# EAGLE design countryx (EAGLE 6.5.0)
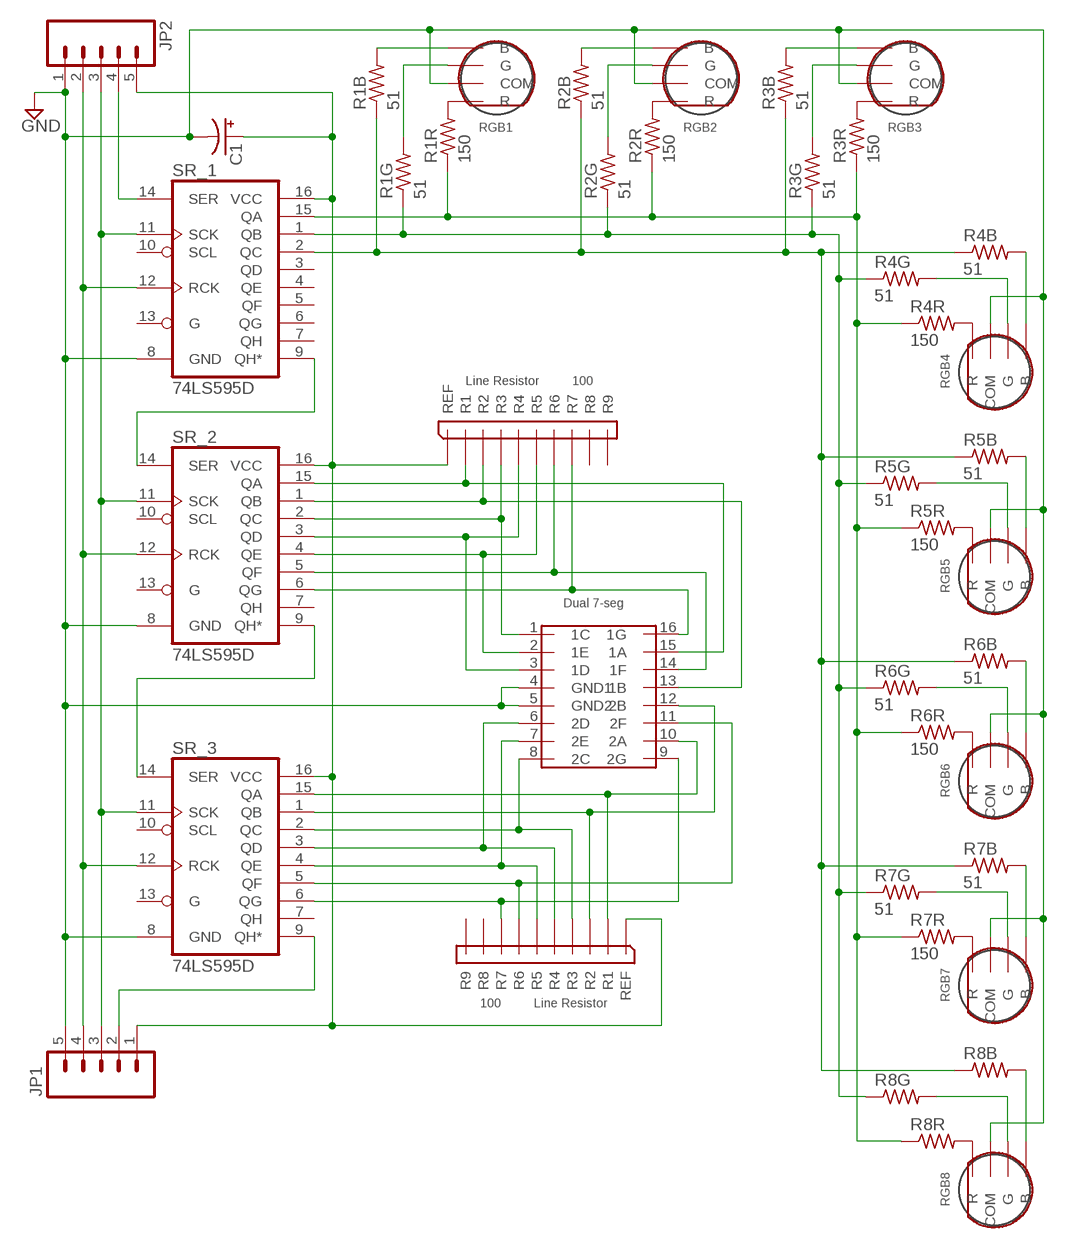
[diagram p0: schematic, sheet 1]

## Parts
C1  CPOL-USE2,5-6E  [E2,5-6E]
JP1  M05LOCK  [1X05_LOCK]
JP2  M05LOCK  [1X05_LOCK]
R1B  51  R-US_0204/5  [0204/5]
R1G  51  R-US_0204/5  [0204/5]
R1R  150  R-US_0204/5  [0204/5]
R2B  51  R-US_0204/5  [0204/5]
R2G  51  R-US_0204/5  [0204/5]
R2R  150  R-US_0204/5  [0204/5]
R3B  51  R-US_0204/5  [0204/5]
R3G  51  R-US_0204/5  [0204/5]
R3R  150  R-US_0204/5  [0204/5]
R4B  51  R-US_0204/5  [0204/5]
R4G  51  R-US_0204/5  [0204/5]
R4R  150  R-US_0204/5  [0204/5]
R5B  51  R-US_0204/5  [0204/5]
R5G  51  R-US_0204/5  [0204/5]
R5R  150  R-US_0204/5  [0204/5]
R6B  51  R-US_0204/5  [0204/5]
R6G  51  R-US_0204/5  [0204/5]
R6R  150  R-US_0204/5  [0204/5]
R7B  51  R-US_0204/5  [0204/5]
R7G  51  R-US_0204/5  [0204/5]
R7R  150  R-US_0204/5  [0204/5]
R8B  R-US_R0805  [R0805]
R8G  R-US_R0805  [R0805]
R8R  R-US_R0805  [R0805]
RGB1  RGBLED  [3LED]
RGB2  RGBLED  [3LED]
RGB3  RGBLED  [3LED]
RGB4  RGBLED  [3LED]
RGB5  RGBLED  [3LED]
RGB6  RGBLED  [3LED]
RGB7  RGBLED  [3LED]
RGB8  RGBLED  [3LED]
SR_1  74LS595D  [SO16]
SR_2  74LS595D  [SO16]
SR_3  74LS595D  [SO16]
U$1  HDSP-G03E  [HDSP-G]
U$2  100  4610X  [4610X]
U$3  100  4610X  [4610X]

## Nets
GND: C1.- JP1.5 JP2.1 RGB1.COM RGB2.COM RGB3.COM RGB4.COM RGB5.COM RGB6.COM RGB7.COM RGB8.COM SR_1.8(GND) SR_2.8(GND) SR_3.8(GND) U$1.4(GND1) U$1.5(GND2)
N$1: R1R.1 R2R.1 R3R.1 R4R.1 R5R.1 R6R.1 R7R.1 R8R.1 SR_1.15(QA)
N$2: R1B.1 R2B.1 R3B.1 R4B.1 R5B.1 R6B.1 R7B.1 R8B.1 SR_1.2(QC)
N$3: R8R.2 RGB8.R
N$4: SR_2.15(QA) U$1.15(1A) U$2.R1
N$5: SR_2.1(QB) U$1.13(1B) U$2.R2
N$6: SR_2.2(QC) U$1.1(1C) U$2.R3
N$7: SR_2.3(QD) U$1.3(1D) U$2.R4
N$8: R1R.2 RGB1.R
N$9: SR_2.5(QF) U$1.14(1F) U$2.R6
N$10: SR_2.6(QG) U$1.16(1G) U$2.R7
N$11: SR_3.6(QG) U$1.9(2G) U$3.R7
N$12: SR_3.5(QF) U$1.11(2F) U$3.R6
N$13: SR_3.4(QE) U$1.7(2E) U$3.R5
N$14: SR_3.3(QD) U$1.6(2D) U$3.R4
N$15: SR_3.2(QC) U$1.8(2C) U$3.R3
N$16: SR_2.4(QE) U$1.2(1E) U$2.R5
N$17: SR_3.15(QA) U$1.10(2A) U$3.R1
N$18: R2R.2 RGB2.R
N$19: SR_3.1(QB) U$1.12(2B) U$3.R2
N$20: R3R.2 RGB3.R
N$25: R1G.2 RGB1.G
N$26: R2G.2 RGB2.G
N$27: R3G.2 RGB3.G
N$28: R1B.2 RGB1.B
N$29: R2B.2 RGB2.B
N$30: R3B.2 RGB3.B
N$32: R1G.1 R2G.1 R3G.1 R4G.1 R5G.1 R6G.1 R7G.1 R8G.1 SR_1.1(QB)
N$34: R4G.2 RGB4.G
N$35: R4B.2 RGB4.B
N$36: R4R.2 RGB4.R
N$39: R5G.2 RGB5.G
N$40: R5B.2 RGB5.B
N$41: R5R.2 RGB5.R
N$43: R6G.2 RGB6.G
N$44: R6B.2 RGB6.B
N$45: R6R.2 RGB6.R
N$46: R8G.2 RGB8.G
N$47: R8B.2 RGB8.B
N$49: R7G.2 RGB7.G
N$50: R7B.2 RGB7.B
N$51: R7R.2 RGB7.R
RCLK: JP1.4 JP2.2 SR_1.12(RCK) SR_2.12(RCK) SR_3.12(RCK)
SCLK: JP1.3 JP2.3 SR_1.11(SCK) SR_2.11(SCK) SR_3.11(SCK)
SER_12: SR_1.9(QH*) SR_2.14(SER)
SER_23: SR_2.9(QH*) SR_3.14(SER)
SER_IN: JP2.4 SR_1.14(SER)
SER_OUT: JP1.2 SR_3.9(QH*)
VCC: C1.+ JP1.1 JP2.5 SR_1.16(VCC) SR_2.16(VCC) SR_3.16(VCC) U$2.REF U$3.REF
Unconnected: SR_1.3(QD) SR_1.4(QE) SR_1.5(QF) SR_1.6(QG) SR_1.7(QH) SR_1.10(SCL) SR_1.13(G) SR_2.7(QH) SR_2.10(SCL) SR_2.13(G) SR_3.7(QH) SR_3.10(SCL) SR_3.13(G) U$2.R8 U$2.R9 U$3.R8 U$3.R9

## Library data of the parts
C1 = Power Supply:CPOL-US: POLARIZED CAPACITOR, American symbol
JP1 JP2 = SparkFun-Connectors:M05: Header 5 Standard 5-pin 0.1" header. Use with straight break away headers (SKU : PRT-00116), right angle break away headers (PRT-00553), swiss pins (PRT-00743), machine pins (PRT-00117), and female headers (PRT-00115). Molex polarized connector foot print use with SKU : PRT-08230 with associated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
R1B R1G R1R R2B R2G R2R R3B R3G R3R R4B R4G R4R R5B R5G R5R R6B R6G R6R R7B R7G R7R R8B R8G R8R = resistor:R-US_: RESISTOR, American symbol
RGB1-RGB8 = RISK:RGBLED
SR_1-SR_3 = SparkFun-DigitalIC:74*595: 8-bit SHIFT REGISTER, output latch; PROD_ID: IC-07875
U$1 = RISK:HDSP-G03E
U$2 U$3 = RISK:4610X

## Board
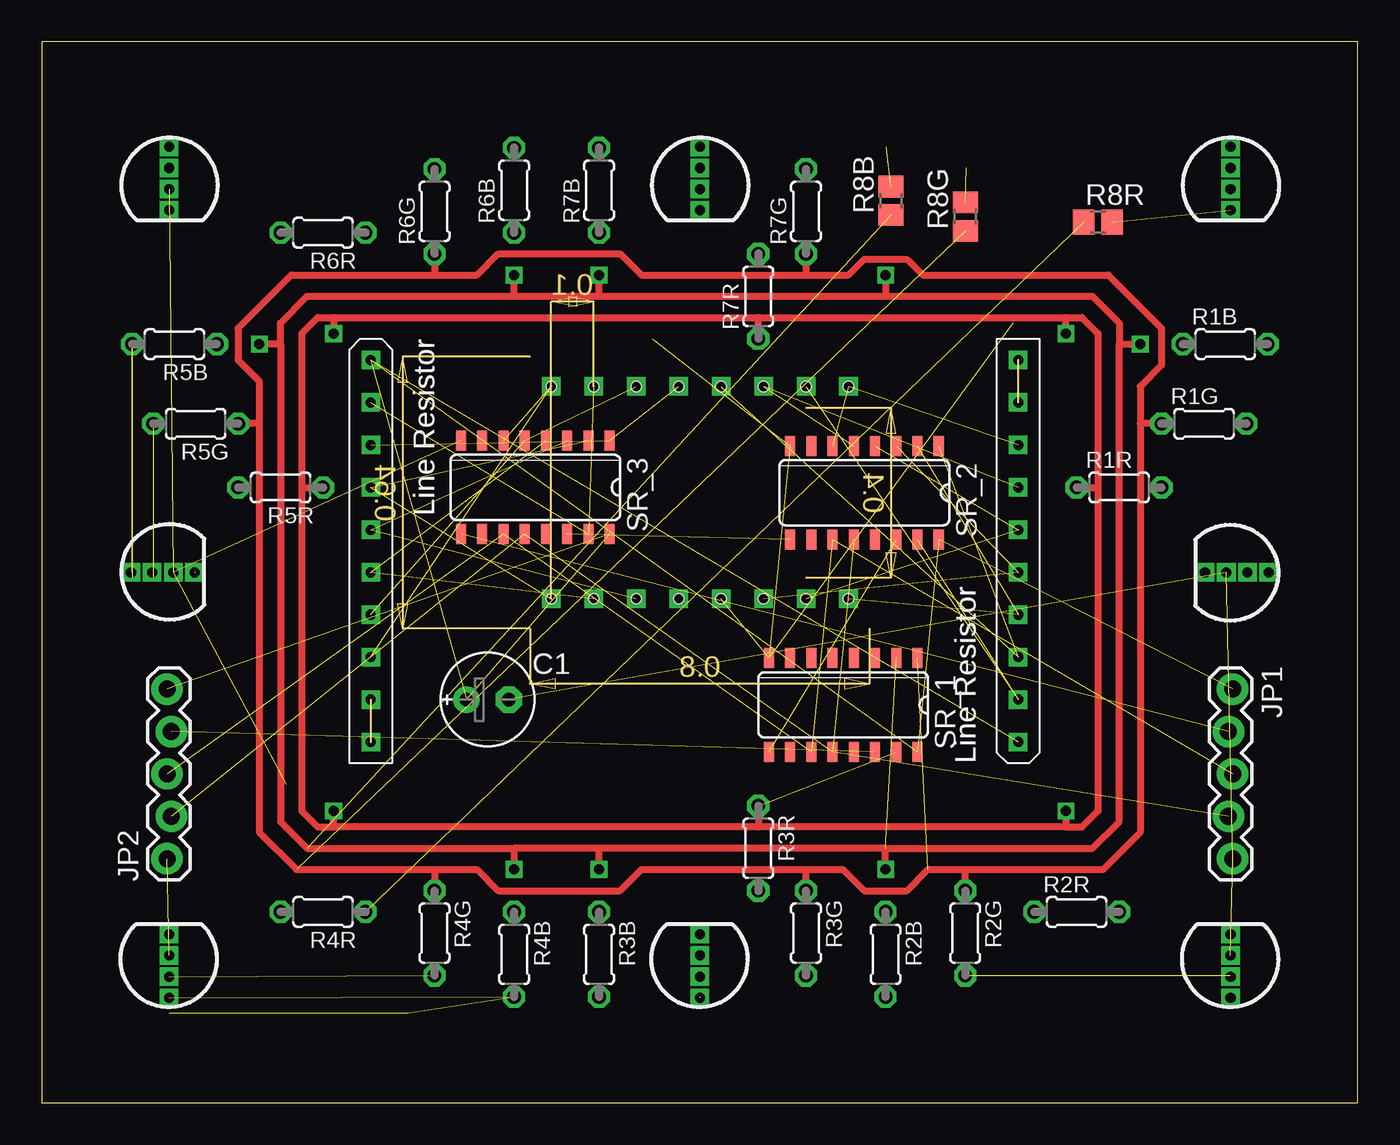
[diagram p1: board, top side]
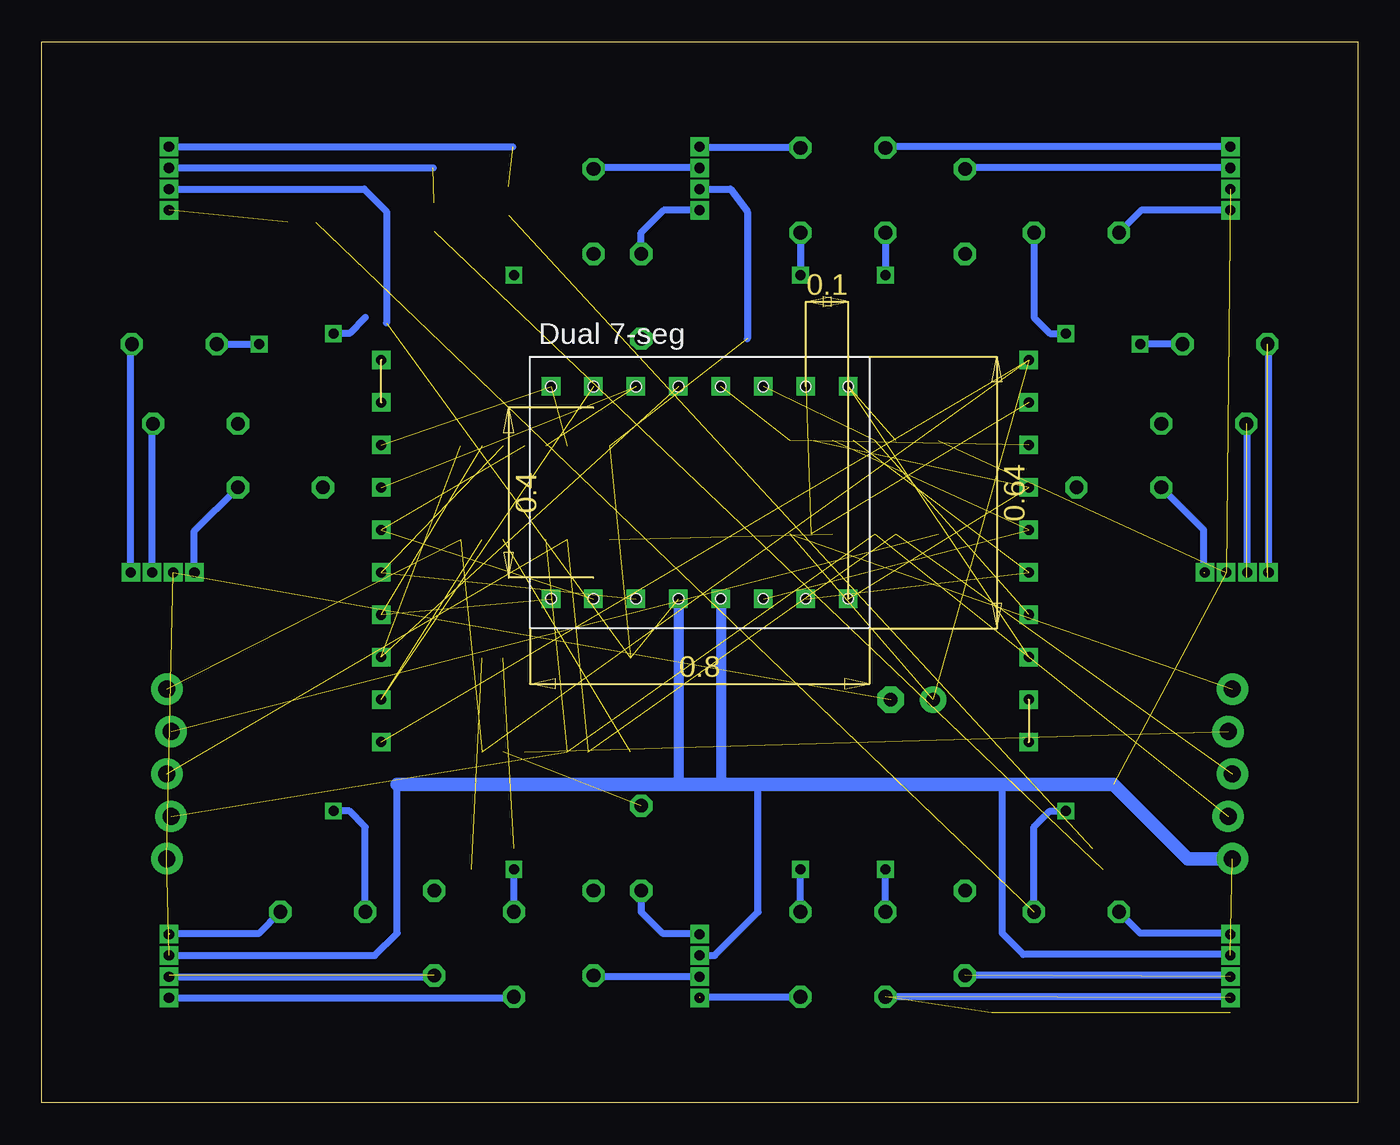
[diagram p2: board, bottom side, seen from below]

Size 78.73 x 63.49 mm. Coordinates in mm from the lower left corner, seen from the top.
Outline: 0,0 78.73,0 78.73,63.49 0,63.49 0,0
Copper layers (1*16): Top 0.035mm / dielectric 1.5mm / Bottom 0.035mm
Design rules "default": minimum track width 10mil, minimum drill 24mil, track to track 8mil, track to pad 8mil, pad to pad 8mil, via to via 8mil, smd to smd 8mil, copper to edge 40mil, drill to drill 8mil, minimum pad ring 10mil, minimum via ring 8mil, stop-mask expansion 4mil, vias tented up to drill 0mil, thermal gap 10mil

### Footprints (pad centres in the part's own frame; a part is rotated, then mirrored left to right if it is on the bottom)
E2,5-6E = drill 0.813 pad 1.575: + -1.27,0 | drill 0.813 pad 1.575 octagon: - 1.27,0
1X05_LOCK = drill 1.016 pad 1.88: 1 0,0.127; 2 2.54,-0.127; 3 5.08,0.127; 4 7.62,-0.127; 5 10.16,0.127
0204/5 = drill 0.813 octagon: 1 -2.54,0; 2 2.54,0
R0805 = smd 1.3 x 1.5: 1 -0.85,0; 2 0.85,0
3LED = drill 0.6 pad 0.61 square: B 0,2.286; COM 0,-0.254; G 0,1.016; R 0,-1.524
SO16 = smd 0.6 x 1.2: 1 -4.445,-2.8; 2 -3.175,-2.8; 3 -1.905,-2.8; 4 -0.635,-2.8; 5 0.635,-2.8; 6 1.905,-2.8; 7 3.175,-2.8; 8 4.445,-2.8; 9 4.445,2.8; 10 3.175,2.8; 11 1.905,2.8; 12 0.635,2.8; 13 -0.635,2.8; 14 -1.905,2.8; 15 -3.175,2.8; 16 -4.445,2.8
HDSP-G = drill 0.6 square: 1 -8.89,-6.35; 2 -6.35,-6.35; 3 -3.81,-6.35; 4 -1.27,-6.35; 5 1.27,-6.35; 6 3.81,-6.35; 7 6.35,-6.35; 8 8.89,-6.35; 9 8.89,6.35; 10 6.35,6.35; 11 3.81,6.35; 12 1.27,6.35; 13 -1.27,6.35; 14 -3.81,6.35; 15 -6.35,6.35; 16 -8.89,6.35 | hole 0.6: 1.27,-6.35; 1.27,-6.35; 1.27,-6.35; 1.27,-6.35; -1.27,-6.35; -1.27,-6.35; -3.81,-6.35; -3.81,-6.35; -6.35,-6.35; -6.35,-6.35; -6.35,-6.35; -8.89,-6.35; -8.89,-6.35; 3.81,-6.35; 3.81,-6.35; 3.81,-6.35; 6.35,-6.35; 6.35,-6.35; 8.89,-6.35; 8.89,-6.35; 8.89,-6.35; 8.89,6.35; 8.89,6.35; 6.35,6.35; 6.35,6.35; 3.81,6.35; 3.81,6.35; 1.27,6.35; 1.27,6.35; -1.27,6.35; -1.27,6.35; -3.81,6.35; -3.81,6.35; -6.35,6.35; -6.35,6.35; -6.35,6.35; -8.89,6.35; -8.89,6.35
4610X = drill 0.6 square: R1 -8.89,0; R2 -6.35,0; R3 -3.81,0; R4 -1.27,0; R5 1.27,0; R6 3.81,0; R7 6.35,0; R8 8.89,0; R9 11.43,0; REF -11.43,0

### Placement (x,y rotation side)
C1  26.67,24.13 0 top
JP1  71.12,24.77 270 top
JP2  7.62,14.61 90 top
R1B  70.8,45.4 0 top
R1G  69.53,40.64 0 top
R1R  64.45,36.83 0 top
R2B  50.48,8.89 270 top
R2G  55.24,10.16 270 top
R2R  61.91,11.43 0 top
R3B  33.34,8.89 270 top
R3G  45.72,10.16 270 top
R3R  42.86,15.24 270 top
R4B  28.26,8.89 270 top
R4G  23.5,10.16 270 top
R4R  16.83,11.43 180 top
R5B  7.94,45.4 180 top
R5G  9.21,40.64 180 top
R5R  14.29,36.83 180 top
R6B  28.26,54.61 90 top
R6G  23.5,53.34 90 top
R6R  16.83,52.07 180 top
R7B  33.34,54.61 90 top
R7G  45.72,53.34 90 top
R7R  42.86,48.26 90 top
R8B  50.8,53.98 90 top
R8G  55.24,53.02 90 top
R8R  63.18,52.7 0 top
RGB1  71.12,31.75 270 top
RGB2  71.12,8.57 180 top
RGB3  39.37,8.57 180 top
RGB4  7.62,8.57 180 top
RGB5  7.62,31.75 90 top
RGB6  7.62,54.93 0 top
RGB7  39.37,54.93 0 top
RGB8  71.12,54.93 0 top
SR_1  47.94,23.81 180 top
SR_2  49.21,36.51 180 top
SR_3  29.53,36.83 180 top
U$1  39.37,36.51 0 bottom
U$2  58.42,33.02 90 top
U$3  19.68,33.02 270 top

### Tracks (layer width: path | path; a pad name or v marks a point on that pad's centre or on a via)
GND  (12 unrouted)
  Bottom 0.406: RGB2.COM 58.8,8.83 57.47,10.16 57.47,19.05 | RGB3.COM 38.48,8.83 35.88,11.43 35.88,19.05 | 21.27,19.05 21.27,10.16 20,8.89 7.62,8.89 | RGB7.COM 37.53,54.67 36.51,53.34 36.51,45.72 | RGB8.COM 59.44,54.67 58.1,53.34 58.1,46.67
  Bottom 0.61: U$1.5 38.1,19.05 | U$1.4 40.64,19.05
  Bottom 0.813: 57.47,19.05 40.64,19.05 38.1,19.05 35.88,19.05 14.61,19.05 10.16,14.61 JP2.1
N$1  (via drill 0.6)  (2 unrouted)
  Top 0.406: 15.56,36.83 15.56,46.04 16.51,46.99 17.46,46.99 | 15.56,36.83 R5R.1 | 15.56,36.83 15.56,17.46 16.51,16.51 17.46,16.51 | 17.46,16.51 v17.46,17.46 | R3R.1 42.86,16.51 | 42.86,16.51 17.46,16.51 | 61.28,16.51 42.86,16.51 | v61.28,17.46 61.28,16.51 | 61.28,16.51 62.23,16.51 63.18,17.46 63.18,36.83 | 17.46,46.99 42.86,46.99 | 42.86,46.99 61.28,46.99 | 61.28,46.99 62.23,46.99 63.18,46.04 63.18,36.83 | v61.28,46.04 61.28,46.99 | R1R.1 63.18,36.83 | R7R.1 42.86,46.99 | 17.46,46.99 v17.46,46.04
  Bottom 0.406: R2R.1 59.37,16.51 60.33,17.46 v61.28,17.46 | R4R.1 19.37,16.51 18.41,17.46 v17.46,17.46 | 59.37,46.99 60.33,46.04 v61.28,46.04 | R6R.1 19.37,46.99 18.41,46.04 v17.46,46.04
N$2  (via drill 0.6)  (2 unrouted)
  Top 0.406: 14.29,45.4 v13.02,45.4 | 14.29,45.4 14.29,16.83 15.88,15.24 28.26,15.24 | 28.26,15.24 v28.26,13.97 | v33.34,13.97 33.34,15.24 | 33.34,15.24 28.26,15.24 | v50.48,13.97 50.48,15.24 | 50.48,15.24 33.34,15.24 | 50.48,15.24 62.87,15.24 64.45,16.83 64.45,45.4 | 14.29,45.4 14.29,46.67 15.88,48.26 28.26,48.26 | 28.26,48.26 33.34,48.26 | 33.34,48.26 50.48,48.26 | 50.48,48.26 62.87,48.26 64.45,46.67 64.45,45.4 | v50.48,49.53 50.48,48.26 | 64.45,45.4 v65.72,45.4 | 33.34,48.26 v33.34,49.53 | 28.26,48.26 v28.26,49.53
  Bottom 0.406: R2B.1 v50.48,13.97 | R3B.1 v33.34,13.97 | R4B.1 v28.26,13.97 | R5B.1 v13.02,45.4 | R1B.1 v65.72,45.4 | R7B.1 v33.34,49.53 | R6B.1 v28.26,49.53
N$3  (1 unrouted)
N$4  (2 unrouted)
N$5  (2 unrouted)
N$6  (2 unrouted)
N$7  (2 unrouted)
N$8
  Bottom 0.406: RGB1.R 69.6,34.23 R1R.2
N$9  (2 unrouted)
N$10  (2 unrouted)
N$11  (2 unrouted)
N$12  (2 unrouted)
N$13  (2 unrouted)
N$14  (2 unrouted)
N$15  (2 unrouted)
N$16  (2 unrouted)
N$17  (2 unrouted)
N$18  (1 unrouted)
  Bottom 0.406: 71.12,10.16 65.72,10.16 R2R.2
N$19  (2 unrouted)
N$20
  Bottom 0.406: R3R.2 42.86,11.43 41.59,10.16 39.43,10.16 RGB3.R
N$25
  Bottom 0.406: RGB1.G 72.14,40.58 R1G.2
N$26  (1 unrouted)
  Bottom 0.406: RGB2.G 55.31,7.56 R2G.2
N$27
  Bottom 0.406: RGB3.G 45.66,7.56 R3G.2
N$28
  Bottom 0.406: RGB1.B 73.41,45.34 R1B.2
N$29
  Bottom 0.406: RGB2.B 50.55,6.29 R2B.2
N$30  (1 unrouted)
  Bottom 0.406: 39.37,6.35 R3B.2
N$32  (2 unrouted)
  Top 0.406: 13.02,40.64 13.02,43.18 11.75,44.45 11.75,46.35 14.92,49.53 23.5,49.53 | 13.02,40.64 R5G.1 | 13.02,40.64 13.02,16.19 15.24,13.97 23.5,13.97 | 23.5,13.97 R4G.1 | 23.5,13.97 26.04,13.97 27.3,12.7 34.61,12.7 35.88,13.97 45.72,13.97 | R3G.1 45.72,13.97 | 45.72,13.97 47.94,13.97 49.21,12.7 51.75,12.7 53.02,13.97 55.24,13.97 | 55.24,13.97 63.5,13.97 65.72,16.19 65.72,40.64 | 45.72,49.53 48.26,49.53 49.21,50.48 51.75,50.48 52.7,49.53 63.82,49.53 66.99,46.35 66.99,44.13 65.72,42.86 65.72,40.64 | R2G.1 55.24,13.97 | R1G.1 65.72,40.64 | R7G.1 45.72,49.53 | R6G.1 23.5,49.53 | 23.5,49.53 26.04,49.53 27.3,50.8 34.61,50.8 35.88,49.53 45.72,49.53
N$34  (1 unrouted)
  Bottom 0.406: 7.62,7.62 R4G.2
N$35  (3 unrouted)
  Bottom 0.406: 7.62,6.35 R4B.2
N$36  (1 unrouted)
  Bottom 0.406: 7.62,10.16 13.02,10.16 R4R.2
N$39  (2 unrouted)
  Bottom 0.406: RGB5.G 6.6,40.58 R5G.2
N$40  (2 unrouted)
  Bottom 0.406: RGB5.B 5.33,45.34 R5B.2
N$41  (1 unrouted)
  Bottom 0.406: 9.21,31.75 9.21,34.29 R5R.2
N$43
  Bottom 0.406: RGB6.G 23.43,55.94 R6G.2
N$44
  Bottom 0.406: RGB6.B 28.19,57.21 R6B.2
N$45
  Bottom 0.406: RGB6.R 12.95,53.4 R6R.2
N$46  (1 unrouted)
  Bottom 0.406: RGB8.G 55.31,55.94
N$47  (1 unrouted)
  Bottom 0.406: RGB8.B 50.55,57.21
N$49
  Bottom 0.406: RGB7.G 45.66,55.94 R7G.2
N$50
  Bottom 0.406: R7B.2 39.31,57.15 RGB7.B
N$51
  Bottom 0.406: RGB7.R 41.53,53.4 42.86,52.07 R7R.2
RCLK  (4 unrouted)
SCLK  (4 unrouted)
SER_12  (1 unrouted)
SER_23  (1 unrouted)
SER_IN  (1 unrouted)
SER_OUT  (1 unrouted)
VCC  (7 unrouted)

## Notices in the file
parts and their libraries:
SparkFun-DigitalIC: Licensing: Creative Commons ShareAlike 4.0 International - https://creativecommons.org/licenses/by-sa/4.0
